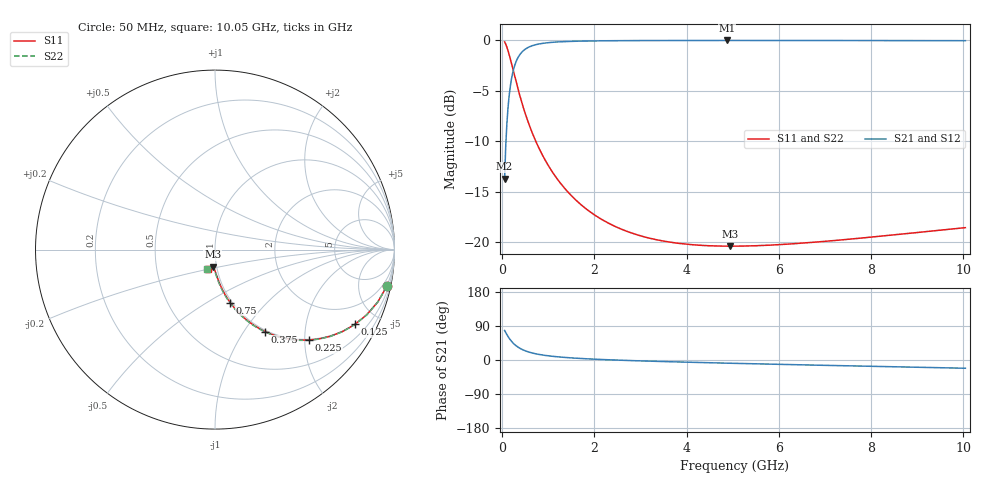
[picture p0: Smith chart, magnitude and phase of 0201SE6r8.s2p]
! AVX Thin Film Operation		Date: August 2001
! Description: Accu-P® Series, Thin Film, SMD, RF Capacitor
! Part Number: 0201ZK6R8BBW
! 50 MHz  -  10.05 GHz
! Serial Measurements
# mhz S db R 50
!	S11		S21		S12		S22
!	dB	Phase	dB	Phase	dB	Phase	dB	Phase
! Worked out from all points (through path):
!   401 points, 50 MHz to 10.05 GHz, reference 50 ohm
!   highest |S21| = -0.05 dB at 4.875 GHz (marker M1); lowest = -13.7 dB at 50 MHz (marker M2)
!   group delay of S21, straight-line fit = 12.2 ps
!   lowest |S11| = -20.4 dB at 4.95 GHz (marker M3), VSWR 1.21, Z = 47.9 - j9.19 ohm
!   |S11| at or under -10 dB: 725.9 MHz to end of sweep
!   |S22| runs from -20.4 to -0.2 dB; largest |S21 - S12| = 0
!   S11 on the Smith chart (normalised r, x): 50 MHz: 0.98, -9.38; 125 MHz: 0.98, -3.75; 225 MHz: 0.98, -2.09; 375 MHz: 0.98, -1.26; 750 MHz: 0.98, -0.64; 10.05 GHz: 0.90, -0.20
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50  -0.19 -12.0  -13.70 77.9  -13.70 77.9  -0.19 -12.1
75  -0.42 -17.8  -10.41 72.2  -10.41 72.2  -0.42 -17.8
125  -1.07 -28.1  -6.63 61.8  -6.63 61.8  -1.07 -28.2
175  -1.89 -36.8  -4.54 53.1  -4.54 53.1  -1.89 -36.9
225  -2.78 -44.0  -3.26 45.9  -3.26 45.9  -2.78 -44.1
300  -4.13 -52.3  -2.13 37.5  -2.13 37.5  -4.13 -52.5
375  -5.41 -58.5  -1.48 31.4  -1.48 31.4  -5.41 -58.7
450  -6.58 -63.2  -1.09 26.7  -1.09 26.7  -6.58 -63.4
525  -7.64 -66.8  -0.83 23.0  -0.83 23.0  -7.64 -67.1
625  -8.89 -70.5  -0.61 19.3  -0.61 19.3  -8.89 -70.8
750  -10.24 -74.0  -0.44 15.8  -0.44 15.8  -10.24 -74.4
950  -12.03 -77.9  -0.29 11.8  -0.29 11.8  -12.03 -78.4
1175  -13.62 -80.9  -0.20 8.7  -0.20 8.7  -13.62 -81.5
1725  -16.34 -85.5  -0.11 3.9  -0.11 3.9  -16.34 -86.4
2475  -18.48 -89.4  -0.07 -0.2  -0.07 -0.2  -18.48 -90.5
3400  -19.79 -92.8  -0.06 -3.8  -0.06 -3.8  -19.79 -94.1
4875  -20.37 -97.2  -0.05 -8.4  -0.05 -8.4  -20.37 -98.6
4950  -20.37 -97.4  -0.05 -8.6  -0.05 -8.6  -20.37 -98.8
5050  -20.37 -97.7  -0.05 -8.9  -0.05 -8.9  -20.37 -99.0
6725  -20.00 -102.2  -0.05 -13.4  -0.05 -13.4  -20.00 -103.4
8400  -19.30 -106.4  -0.06 -17.6  -0.06 -17.6  -19.30 -107.5
10050  -18.54 -110.5  -0.07 -21.7  -0.07 -21.7  -18.54 -111.5
